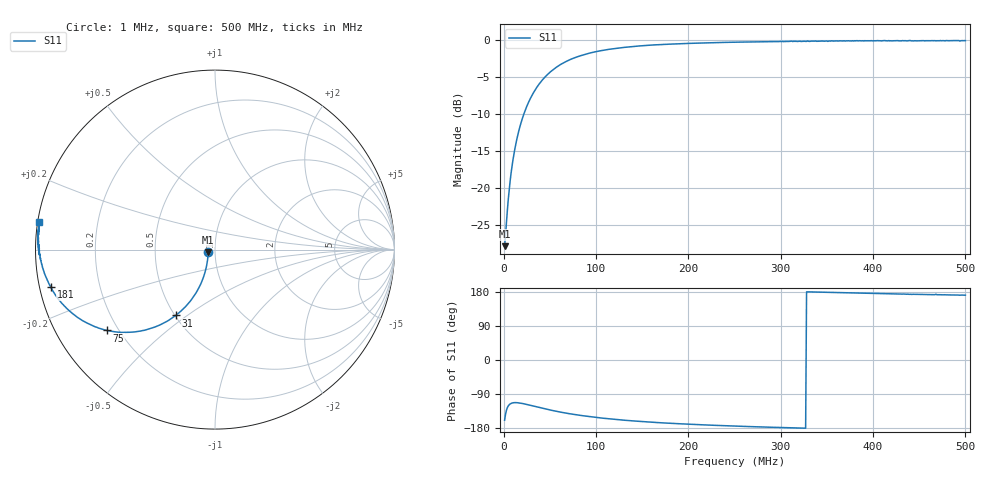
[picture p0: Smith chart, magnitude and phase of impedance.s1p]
# Hz S RI R 50.0
! written by SimSmith version 18.3b
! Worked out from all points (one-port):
!   500 points, 1 MHz to 500 MHz, reference 50 ohm
!   lowest |S11| = -27.8 dB at 1 MHz (marker M1), VSWR 1.08, Z = 46.3 - j1.37 ohm
!   |S11| at or under -10 dB: start of sweep to 21.79 MHz
!   S11 on the Smith chart (normalised r, x): 1 MHz: 0.93, -0.03; 31 MHz: 0.50, -0.45; 75 MHz: 0.16, -0.33; 181 MHz: 0.03, -0.11; 500 MHz: 0.00, +0.08
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1000000  -0.038 -0.0148
2000000  -0.0388 -0.0291
3000000  -0.0401 -0.0437
5000000  -0.0436 -0.0725
7000000  -0.0491 -0.1009
8000000  -0.0527 -0.115
1e7  -0.0605 -0.1425
1.3e7  -0.0753 -0.1821
1.7e7  -0.1001 -0.2317
2.1e7  -0.1301 -0.2771
2.6e7  -0.1727 -0.3261
3.1e7  -0.219 -0.367
3.8e7  -0.2877 -0.4104
4.7e7  -0.3751 -0.4444
5.5e7  -0.4482 -0.4587
6.4e7  -0.5228 -0.4615
7.5e7  -0.6021 -0.4506
8.7e7  -0.6721 -0.4282
1e8  -0.7339 -0.3982
1.26e8  -0.8203 -0.3325
1.52e8  -0.8763 -0.2713
1.81e8  -0.9145 -0.2101
1.89e8  -0.9222 -0.1952
2.51e8  -0.9624 -0.0943
3.13e8  -0.977 -0.019
3.76e8  -0.9851 0.0502
4.38e8  -0.9825 0.1076
5e8  -0.9781 0.1543
